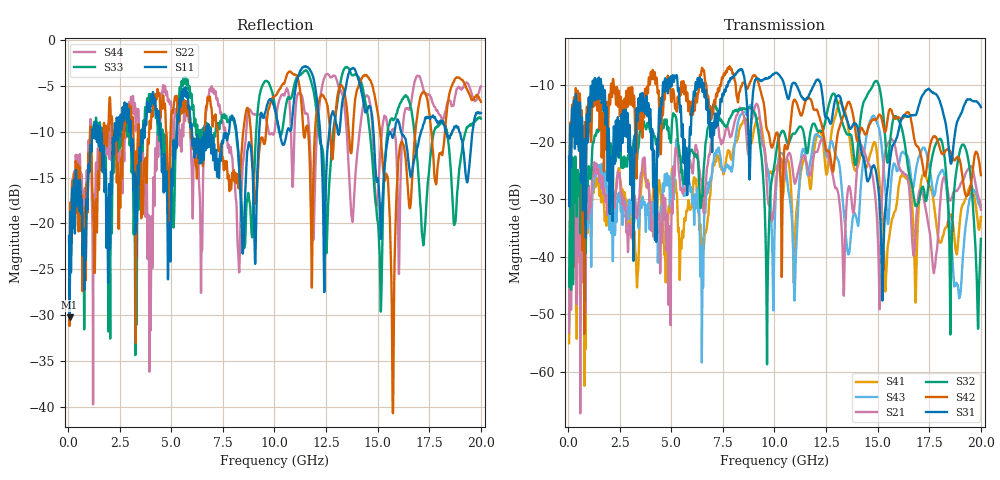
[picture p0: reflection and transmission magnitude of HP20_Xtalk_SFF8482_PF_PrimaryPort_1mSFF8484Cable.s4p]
# MHz S MA R 50.00
! FREQ  S11  S12  S13  S14
!  S21  S22  S23  S24
!  S31  S32  S33  S34
!  S41  S42  S43  S44
!  MAG  ANG  MAG  ANG  MAG  ANG  MAG  ANG
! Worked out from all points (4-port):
!   1996 points, 50 MHz to 20 GHz, reference 50 ohm
!   strongest paths, dB at 50 MHz, 5.04 GHz, 10.03 GHz, 15.02 GHz, 20 GHz:
!     S31: -22.5, -9.4, -8.0, -27.7, -13.9
!     S42: -22.7, -12.0, -19.1, -15.6, -25.8
!     S32: -45.2, -16.3, -23.1, -9.8, -36.9
!     S21: -53.2, -31.1, -28.9, -37.7, -31.8
!     S43: -52.1, -26.9, -32.2, -17.1, -31.0
!     S41: -55.1, -24.6, -24.8, -24.2, -33.1
!   lowest |S11| = -30.2 dB at 70 MHz (marker M1), VSWR 1.06, Z = 52.9 - j1.33 ohm
!   |S11| at or under -10 dB: start of sweep to 1.162 GHz; 8.154 GHz to 9.258 GHz (1.104 GHz wide, 12.7 % of centre); 14.79 GHz to 15.82 GHz (1.027 GHz wide, 6.71 % of centre)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
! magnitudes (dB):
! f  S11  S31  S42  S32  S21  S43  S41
! 50 MHz  -21.4  -22.5  -22.7  -45.2  -53.2  -52.1  -55.1
! 70 MHz  -30.2  -31.3  -29.6  -37.3  -42.2  -42.5  -44.4
! 8.34 GHz  -16.2  -7.3  -10.8  -14.3  -14.0  -15.4  -17.3
! 9.64 GHz  -7.1  -9.0  -17.9  -58.7  -28.0  -24.4  -25.3
! 14.92 GHz  -14.8  -25.2  -16.1  -9.4  -31.0  -16.2  -20.8
! 15.73 GHz  -10.7  -20.6  -15.2  -16.4  -19.7  -24.5  -33.1
! 20 GHz  -8.0  -13.9  -25.8  -36.9  -31.8  -31.0  -33.1
